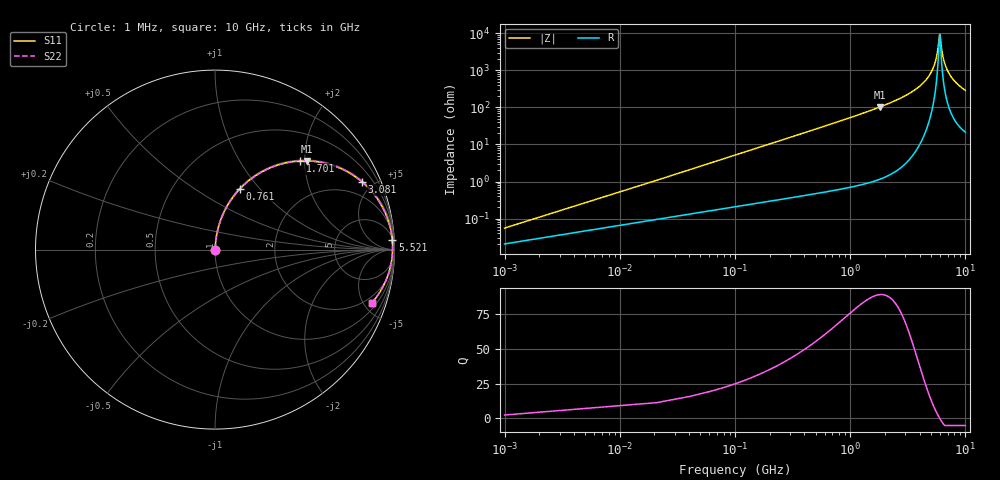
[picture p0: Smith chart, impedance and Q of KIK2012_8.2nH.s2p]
!version-2
!date-01.2022
!Series
# MHz S RI R 50
!Freq ReS11 ImS11 ReS21 ImS21 ReS12 ImS12 ReS22 ImS22
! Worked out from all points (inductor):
!   501 points, 1 MHz to 10 GHz, reference 50 ohm
!   read as one part in series: L = 8.2 nH near 41 MHz
!   highest Q = 88.9 at 1.801 GHz (marker M1), where L = 9.01 nH
!   self-resonance near 5.981 GHz
!   S11 on the Smith chart (normalised r, x): 1 MHz: 1.00, +0.00; 761 MHz: 1.01, +0.80; 1.701 GHz: 1.02, +1.91; 3.081 GHz: 1.06, +4.32; 5.521 GHz: 8, +36; 10 GHz: 1.43, -5.76
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1  0.000207 0.000515  0.9998 -0.000515  0.9998 -0.000515  0.000207 0.000515
61  0.0026 0.0313  0.9974 -0.0313  0.9974 -0.0313  0.0026 0.0313
101  0.00476 0.0517  0.9952 -0.0517  0.9952 -0.0517  0.00476 0.0517
161  0.00942 0.082  0.9906 -0.082  0.9906 -0.082  0.00942 0.082
381  0.041 0.1882  0.959 -0.1882  0.959 -0.1882  0.041 0.1882
761  0.1407 0.3404  0.8593 -0.3404  0.8593 -0.3404  0.1407 0.3404
1681  0.4695 0.4934  0.5305 -0.4934  0.5305 -0.4934  0.4695 0.4934
1701  0.4764 0.4938  0.5236 -0.4938  0.5236 -0.4938  0.4764 0.4938
1801  0.5099 0.4943  0.4901 -0.4943  0.4901 -0.4943  0.5099 0.4943
3081  0.8196 0.3771  0.1804 -0.3771  0.1804 -0.3771  0.8196 0.3771
3341  0.8576 0.341  0.1424 -0.341  0.1424 -0.341  0.8576 0.341
4301  0.9479 0.2058  0.0521 -0.2058  0.0521 -0.2058  0.9479 0.2058
5001  0.9782 0.1143  0.0218 -0.1143  0.0218 -0.1143  0.9782 0.1143
5521  0.9878 0.052  0.0122 -0.052  0.0122 -0.052  0.9878 0.052
5701  0.9891 0.0317  0.0109 -0.0317  0.0109 -0.0317  0.9891 0.0317
5941  0.9895 0.00555  0.0105 -0.00555  0.0105 -0.00555  0.9895 0.00555
6001  0.9894 -0.000821  0.0106 0.000821  0.0106 0.000821  0.9894 -0.000821
6321  0.9874 -0.0336  0.0126 0.0336  0.0126 0.0336  0.9874 -0.0336
6681  0.9828 -0.0684  0.0172 0.0684  0.0172 0.0684  0.9828 -0.0684
7341  0.969 -0.1262  0.031 0.1262  0.031 0.1262  0.969 -0.1262
8341  0.939 -0.2007  0.061 0.2007  0.061 0.2007  0.939 -0.2007
10000  0.8755 -0.2949  0.1245 0.2949  0.1245 0.2949  0.8755 -0.2949
